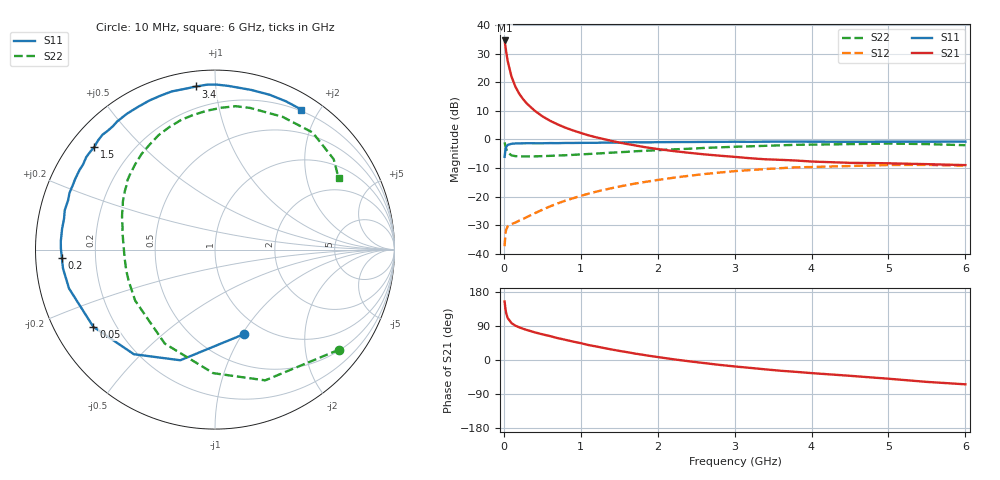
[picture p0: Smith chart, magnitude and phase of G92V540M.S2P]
! SIEMENS Small Signal Semiconductors
! BFG235
! Si NPN RF Bipolar Junction Transistor in SOT223
! VCE = 2.5 V  IC = 40 mA
! Common Emitter S-Parameters:  July  1994
# GHz  S  MA  R  50
!  f  S11  S21  S12  S22
! GHz  MAG  ANG  MAG  ANG  MAG  ANG  MAG  ANG
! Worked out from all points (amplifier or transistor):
!   40 points, 10 MHz to 6 GHz, reference 50 ohm
!   highest |S21| = 34.6 dB at 10 MHz (marker M1)
!   |S21| within 3 dB of that: start of sweep to 25.75 MHz
!   unconditionally stable (mu >= 1): 495.9 MHz to 1.506 GHz
!   at 200 MHz: K = 0.63, MSG = 22.2 dB, |S12| = -28.4 dB
!   at 1.5 GHz: K = 1.00, MAG = 7.4 dB, |S12| = -16.4 dB
!   at 6 GHz: K = 0.94, MSG = 0.1 dB, |S12| = -9.1 dB
!   S11 on the Smith chart (normalised r, x): 10 MHz: 0.81, -1.01; 50 MHz: 0.12, -0.29; 200 MHz: 0.08, -0.03; 1.5 GHz: 0.07, +0.37; 3.4 GHz: 0.08, +0.89; 6 GHz: 0.18, +1.78
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0.01  0.4981 -71.4  53.67 154.5  0.0137 66.3  0.8887 -38.8
0.02  0.6461 -107.4  43.2 136.1  0.0221 49.8  0.7803 -69.0
0.03  0.7376 -127.8  34.55 124.0  0.0266 40.5  0.6885 -90.8
0.05  0.8029 -147.6  23.39 110.7  0.0304 30.4  0.5937 -118.1
0.1  0.8417 -165.1  12.46 97.3  0.0334 26.5  0.5279 -147.4
0.15  0.8533 -172.9  8.388 90.6  0.0354 29.2  0.5119 -159.8
0.2  0.8543 -176.9  6.291 86.2  0.0382 32.9  0.5081 -166.7
0.25  0.8586 179.7  5.069 82.4  0.0411 36.3  0.5054 -171.3
0.3  0.8605 177.0  4.232 79.2  0.0441 39.1  0.506 -174.9
0.4  0.8597 172.3  3.189 73.1  0.0514 44.0  0.5075 180.0
0.5  0.8586 168.4  2.547 67.8  0.0592 46.9  0.5122 175.9
0.6  0.8654 165.3  2.128 63.1  0.0678 48.6  0.5178 172.4
0.7  0.8634 161.4  1.833 57.7  0.0765 49.6  0.5251 169.1
0.9  0.8697 155.8  1.438 48.6  0.0942 49.5  0.5392 163.5
1.1  0.8754 149.4  1.182 39.5  0.113 47.9  0.5582 157.8
1.5  0.8831 139.6  0.884 24.1  0.1505 42.3  0.5996 146.8
2.2  0.9022 122.9  0.629 2.0  0.2142 28.4  0.6716 127.5
3.2  0.9112 101.0  0.471 -20.8  0.2924 5.0  0.7601 99.2
3.4  0.9148 96.6  0.451 -24.7  0.3044 0.1  0.7754 93.2
4.5  0.9122 77.2  0.391 -41.7  0.3441 -25.6  0.8301 63.0
5.5  0.9159 64.4  0.371 -57.8  0.36 -47.6  0.8313 37.3
6  0.9167 58.3  0.357 -64.2  0.3491 -55.8  0.795 29.9
